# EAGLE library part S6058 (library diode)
Si PIN Quadrant photodiode Source: http://sales.hamamatsu.com/assets/pdf/parts_S/S7379-01_etc.pdf
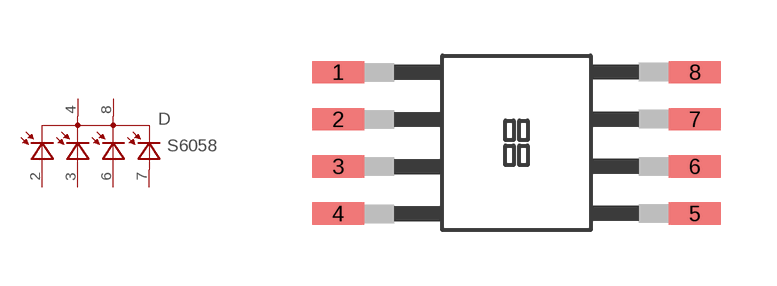
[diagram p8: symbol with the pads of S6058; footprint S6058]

Designator prefix D

## S6058  [S6058]
2  AA  pas
3  AB  pas
4  C1  pas
6  AC  pas
7  AD  pas
8  C2  pas

## Footprint S6058 (pad centres in mm)
Si PIN Quadrant photodiode Source: http://sales.hamamatsu.com/assets/pdf/parts_S/S7379-01_etc.pdf
smd 1.4 x 0.6: 1 -4.805,1.905; 2 -4.805,0.635; 3 -4.805,-0.635; 4 -4.805,-1.905; 5 4.805,-1.905; 6 4.805,-0.635; 7 4.805,0.635; 8 4.805,1.905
